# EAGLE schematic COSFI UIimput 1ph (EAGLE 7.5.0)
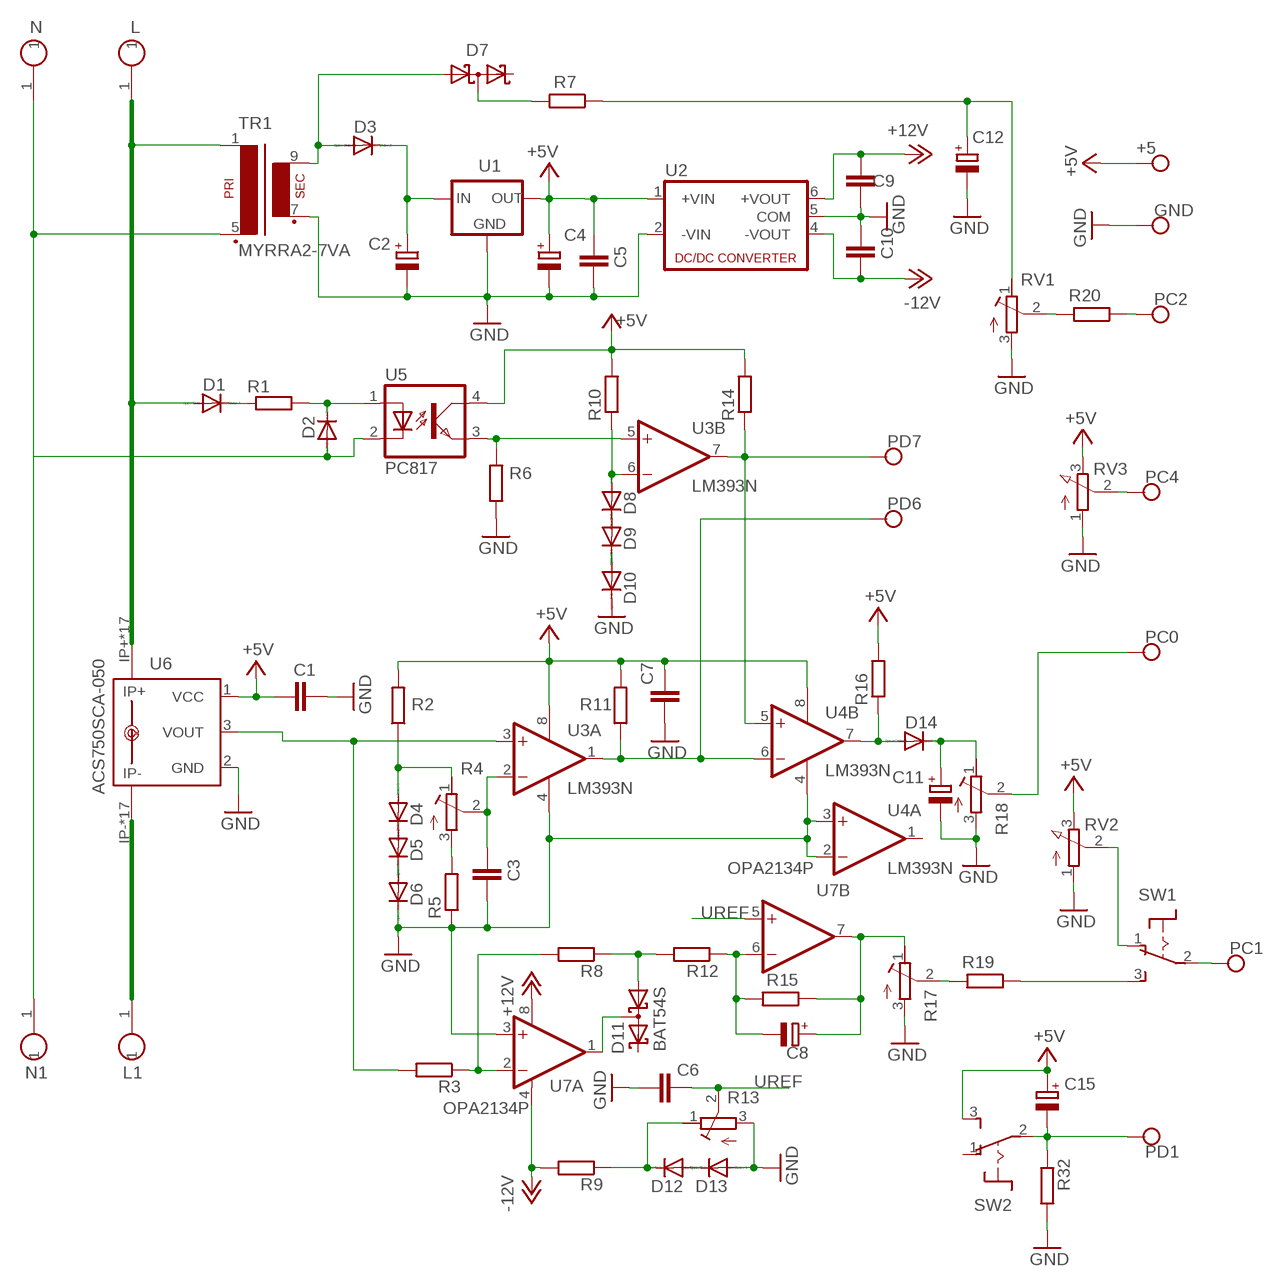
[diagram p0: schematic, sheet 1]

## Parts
+5  CONNWIRE  [CONNWIRE]
C1  C-EUC1206  [C1206]
C2  CPOL-EUE5-8.5  [E5-8,5]
C3  C-EUC1206  [C1206]
C4  CPOL-EUE2-5  [E2-5]
C5  C-EUC1206  [C1206]
C6  C-EUC1206  [C1206]
C7  C-EUC1206  [C1206]
C8  CPOL-EUE2-5  [E2-5]
C9  C-EUC1206  [C1206]
C10  C-EUC1206  [C1206]
C11  CPOL-EUE2-5  [E2-5]
C12  CPOL-EUE3.5-8  [E3,5-8]
C15  CPOL-EUE2-5  [E2-5]
D1  1N4004  [DO41-10]
D2  1N4004  [DO41-10]
D3  1N4004  [DO41-10]
D4  1N4148DO35-7  [DO35-7]
D5  1N4148DO35-7  [DO35-7]
D6  1N4148DO35-7  [DO35-7]
D7  BAT54S  [SOT23]
D8  1N4148DO35-7  [DO35-7]
D9  1N4148DO35-7  [DO35-7]
D10  1N4148DO35-7  [DO35-7]
D11  BAT54S  [SOT23]
D12  1N4148DO35-7  [DO35-7]
D13  1N4148DO35-7  [DO35-7]
D14  1N4148DO35-7  [DO35-7]
GND  CONNWIRE  [CONNWIRE]
L  CONNHOLE  [CONNHOLE4]
L1  CONNHOLE  [CONNHOLE4]
N  CONNHOLE  [CONNHOLE4]
N1  CONNHOLE  [CONNHOLE4]
PC0  CONNWIRE  [CONNWIRE]
PC1  CONNWIRE  [CONNWIRE]
PC2  CONNWIRE  [CONNWIRE]
PC4  CONNWIRE  [CONNWIRE]
PD1  CONNWIRE  [CONNWIRE]
PD6  CONNWIRE  [CONNWIRE]
PD7  CONNWIRE  [CONNWIRE]
R1  R-EU_0617/22  [0617/22]
R2  R-EU_0204/7  [0204/7]
R3  R-EU_0204/7  [0204/7]
R4  R-TRIMM-3386-F  [R-TRIMM-3386F]
R5  R-EU_0204/7  [0204/7]
R6  R-EU_0204/7  [0204/7]
R7  R-EU_0204/7  [0204/7]
R8  R-EU_0204/7  [0204/7]
R9  R-EU_0204/7  [0204/7]
R10  R-EU_0204/7  [0204/7]
R11  R-EU_0204/7  [0204/7]
R12  R-EU_0204/7  [0204/7]
R13  R-TRIMM-3386-F  [R-TRIMM-3386F]
R14  R-EU_0204/7  [0204/7]
R15  R-EU_0204/7  [0204/7]
R16  R-EU_0204/7  [0204/7]
R17  R-TRIMM-3386-F  [R-TRIMM-3386F]
R18  R-TRIMM-3386-F  [R-TRIMM-3386F]
R19  R-EU_0204/7  [0204/7]
R20  R-EU_0204/7  [0204/7]
R32  R-EU_0204/7  [0204/7]
RV1  R-TRIMM-3386-F  [R-TRIMM-3386F]
RV2  PTV09A  PV09A  [PTV09]
RV3  PTV09A  PV09A  [PTV09]
SW1  8MS9P1  [8MS9]
SW2  8MS9P1  [8MS9]
TR1  MYRRA2-7VA  [MYRRA2-7]
U1  78XXL  [78XXL]
U2  NMA  [NMA]
U3  LM393N  [DIL08]
U4  LM393N  [DIL08]
U5  PC817  [DIL04]
U6  ACS750SCA-050  [ACS75050]
U7  OPA2134P  [DIL08]

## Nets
+5V: +5.P$1 C1.2 C4.+ C5.1 C7.2 C15.+ R2.2 R10.2 R11.2 R14.2 R16.2 RV2.3(E) RV3.3(E) SW2.3(S) U1.OUT U2.1(+VIN) U3.8(P:V+) U4.8(P:V+) U5.4(COL) U6.1(VCC)
+12V: C9.1 U2.6(+VOUT) U7.8(A:V+)
-12V: C10.2 R9.2 U2.4(-VOUT) U7.4(A:V-)
GND: C1.1 C2.- C3.2 C4.- C5.2 C6.1 C7.1 C9.2 C10.1 C11.- C12.- D6.C D10.C D13.A GND.P$1 R5.1 R6.1 R13.3(E) R17.3(E) R18.3(E) R32.2 RV1.3(E) RV2.1(A) RV3.1(A) TR1.7(S3) U1.GND U2.2(-VIN) U2.5(COM) U3.4(P:V-) U4.2(A:-IN) U4.3(A:+IN) U4.4(P:V-) U6.2(GND) U7.3(A:+IN)
N$1: D1.C R1.1
N$2: R3.1 R8.2 U7.2(A:-IN)
N$3: D2.C R1.2 U5.1(A)
N$4: D8.C D9.A
N$5: D2.A N1.1 N.1 TR1.5(P2) U5.2(C)
N$6: D1.A L.1 TR1.1 U6.IP+ U6.IP+@2(IP+) U6.IP+@3(IP+) U6.IP+@4(IP+) U6.IP+@5(IP+) U6.IP+@6(IP+) U6.IP+@7(IP+) U6.IP+@8(IP+) U6.IP+@9(IP+) U6.IP+@10(IP+) U6.IP+@11(IP+) U6.IP+@12(IP+) U6.IP+@13(IP+) U6.IP+@14(IP+) U6.IP+@15(IP+) U6.IP+@16(IP+) U6.IP+@17(IP+)
N$7: RV2.2(S) SW1.1(O)
N$8: D9.C D10.A
N$9: D12.A D13.C
N$10: D12.C R9.1 R13.1(A)
N$11: R4.3(E) R5.2
N$12: D4.A R2.1 R4.1(A)
N$13: R6.2 U3.5(B:+IN) U5.3(EMIT)
N$14: R3.2 U3.3(A:+IN) U6.3(VOUT)
N$15: D4.C D5.A
N$16: D8.A R10.1 U3.6(B:-IN)
N$17: D14.A R16.1 U4.7(B:OUT)
N$18: PD7.P$1 R14.1 U3.7(B:OUT) U4.5(B:+IN)
N$19: D5.C D6.A
N$20: PD6.P$1 R11.1 U3.1(A:OUT) U4.6(B:-IN)
N$21: C3.1 R4.2(S) U3.2(A:-IN)
N$22: C11.+ D14.C R18.1(A)
N$23: PC0.P$1 R18.2(S)
N$24: D11.3(C1A2) U7.1(A:OUT)
N$25: PC1.P$1 SW1.2(P)
N$26: PC4.P$1 RV3.2(S)
N$27: R19.1 SW1.3(S)
N$28: PC2.P$1 R20.1
N$29: D3.A D7.1(A1) TR1.9(S4)
N$30: D7.3(C1A2) R7.2
N$31: D11.1(A1) R8.1 R12.2
N$32: C8.- R12.1 R15.2 U7.6(B:-IN)
N$33: C8.+ R15.1 R17.1(A) U7.7(B:OUT)
N$34: C15.- PD1.P$1 R32.1 SW2.2(P)
N$35: R17.2(S) R19.2
N$37: C2.+ D3.C U1.IN
N$38: R20.2 RV1.2(S)
N$40: C12.+ R7.1 RV1.1(A)
N$41: L1.1 U6.IP- U6.IP-@2(IP-) U6.IP-@3(IP-) U6.IP-@4(IP-) U6.IP-@5(IP-) U6.IP-@6(IP-) U6.IP-@7(IP-) U6.IP-@8(IP-) U6.IP-@9(IP-) U6.IP-@10(IP-) U6.IP-@11(IP-) U6.IP-@12(IP-) U6.IP-@13(IP-) U6.IP-@14(IP-) U6.IP-@15(IP-) U6.IP-@16(IP-) U6.IP-@17(IP-)
UREF: C6.2 R13.2(S) U7.5(B:+IN)
Unconnected: D7.2(C2) D11.2(C2) SW2.1(O) U4.1(A:OUT)

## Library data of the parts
+5 GND PC0 PC1 PC2 PC4 PD1 PD6 PD7 = connholes:CONNWIRE
C1 C3 C5-C7 C9 C10 = rcl:C-EU: CAPACITOR, European symbol
C2 C4 C8 C11 C12 C15 = rcl:CPOL-EU: POLARIZED CAPACITOR, European symbol
D1-D3 = diode:1N4004: DIODE
D4-D6 D8-D10 D12-D14 = diode:1N4148: DIODE
D7 D11 = diode:BAT54S: Schottky Diodes Pin connection corrected 2011-05-04 Source: Fairchild .. BAT54.pdf
L L1 N N1 = connholes:CONNHOLE
R1-R3 R5-R12 R14-R16 R19 R20 R32 = rcl:R-EU_: RESISTOR, European symbol
R4 R13 R17 R18 RV1 = rcl:R-TRIMM-3386-F
RV2 RV3 = pot:PV09A
SW1 SW2 = switch:8MS9P1
TR1 = trafo:MYRRA2-7VA
U1 = v-reg:78XXL: VOLTAGE REGULATOR
U2 = dc-dc-converter:NMA: DC-DC CONVERTER; MF: C & D TECHNOLOGIES, INC; MPN: NMA0515SC; OC_FARNELL: 1021434; OC_NEWARK: 61K3064
U3 U4 = linear:LM393: COMPARATOR
U5 = optocoupler:PC817: SHARP OPTO COUPLER; MPN: PC817X4J000F; OC_FARNELL: 9707727; OC_NEWARK: 97K7059
U6 = allegro:ACS750*CA-050: Current Sensor display layer 49 Reference in BRD and place VIAs on circles Source: www.allegromicro.com/datafile/0750-050.pdf; MF: ALLEGRO MICROSYSTEMS, INC.; MPN: ACS750SCA-050; OC_FARNELL: 1457175; OC_NEWARK: 81H6588
U7 = burr-brown:OPA2134: Operational Amplifier; MF: TEXAS INSTRUMENTS; MPN: OPA2134PA; OC_FARNELL: 1097574; OC_NEWARK: 74K3897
